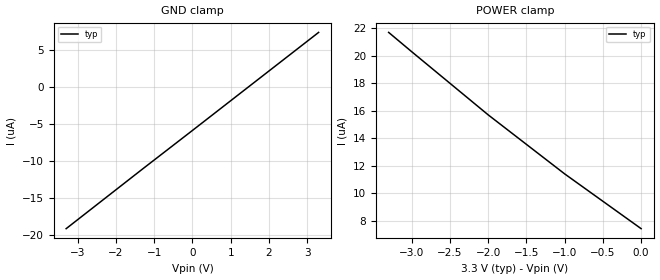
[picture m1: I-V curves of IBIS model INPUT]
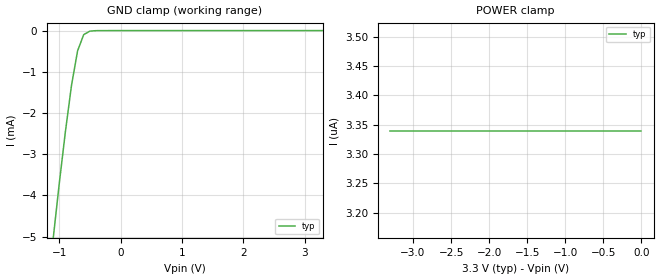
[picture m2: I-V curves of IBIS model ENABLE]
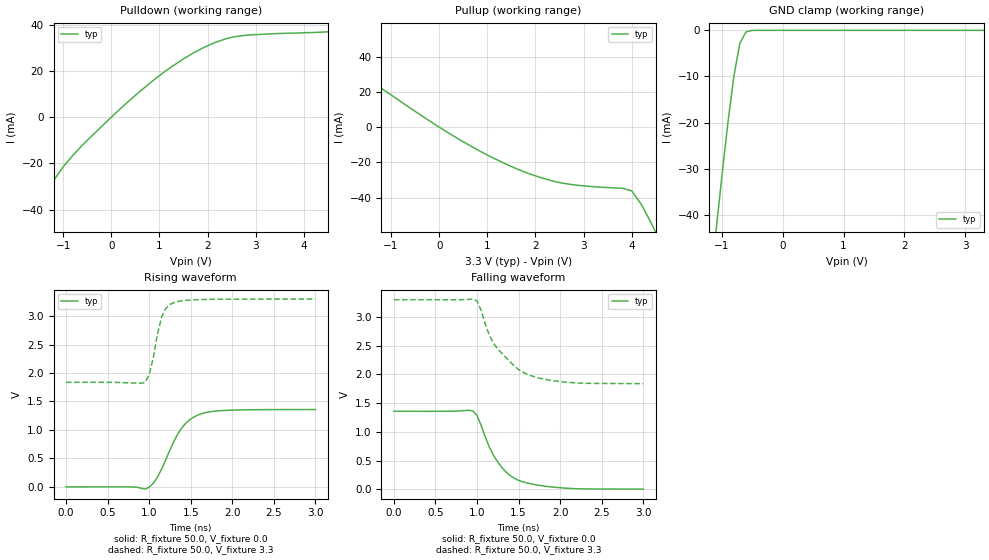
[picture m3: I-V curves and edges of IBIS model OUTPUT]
|   Texas Instruments Incorporated
|   Data Transmissions Products
|   IBIS Model for SN65LVDS352
|   24PW TSSOP Package
[IBIS Ver]   3.2
[Comment char]   |_char
[File name]   lvds352.ibs
[File Rev]   1.0
[Date]   23Aug01
[Source]   File originated at Texas Instruments Incorporated.
   Data Transmission Products Group. All data based on
   Bench Measurements.
[Notes]
[Disclaimer]
(C) Copyright Texas Instruments Incorporated 2001
   All rights reserved
  Texas Instruments Incorporated hereby grants the user of this IBIS
model a non-exclusive, nontransferable license to use this IBIS model
under the following terms.  Before using this IBIS model, the user
should read this license.  If the user does not accept these terms,
the IBIS model should be returned to Texas Instruments within 30 days.
  The user is granted this license only to use the IBIS model and
is not granted rights to sell, load, rent, lease or license the IBIS
model in whole or in part, or in modified form to anyone other than
user.  User may modify the IBIS model to suit its specific applications
but rights to derivative works and such modifications shall belong to
Texas Instruments.
  This IBIS model is provided on an "AS IS" basis and Texas Instruments
makes absolutely no warranty with respect to the information contained
herein.  TEXAS INSTRUMENTS DISCLAIMS AND CUSTOMER WAIVES ALL WARRANTIES,
EXPRESS OR IMPLIED, INCLUDING WARRANTIES OF MERCHANTABILITY OR FITNESS
FOR A PARTICULAR PURPOSE. The entire risk as to quality and performance
is with the Customer. ACCORDINGLY, IN NO EVENT SHALL THE COMPANY BE LIABLE
FOR ANY DAMAGES, WHETHER IN CONTRACT OR TORT,INCLUDING ANY LOST PROFITS
OR OTHER INCIDENTAL, CONSEQUENTIAL, EXEMPLARY, OR PUNITIVE DAMAGES ARISING
OUT OF THE USE OR APPLICATION OF THE IBIS model provided in this package.
Further, Texas Instruments reserves the right to discontinue or make changes
without notice to any product herein to improve reliability, function, or
design. Texas Instruments does not convey any license under patent rights
or any other intellectual property rights, including those of third parties.
Contact Texas Instruments at ATTN:DATA TRANSMISSIONS
[Copyright]   Copyright 2001, Texas Instruments, All Rights Reserved
[Component]   SN65LVDS352PW
[Manufacturer]  Texas Instruments Incorporated
[Package]
|   typ   min   max
R_pkg   0.039   0.030   0.046
L_pkg   2.685nH   2.367nH   3.177nH
C_pkg   0.320pF   0.252pF   0.434pF
[Pin]   signal_name   model_name   R_pin   L_pin   C_pin
1   1A   INPUT   0.037   3.153n   0.434p
2   1B   INPUT   0.034   2.629n   0.341p
3   2A   INPUT   0.032   2.860n   0.347p
4   2B   INPUT   0.042   2.741n   0.290p
5   EN1,2   ENABLE   0.046   2.600n   0.262p
6   VCC   POWER   0.043   2.414n   0.266p
7   GND   GND   0.042   2.367n   0.262p
8   EN3,4   ENABLE   0.044   2.461n   0.252p
9   3A   INPUT   0.042   2.543n   0.274p
10   3B   INPUT   0.030   2.616n   0.332p
11   4A   INPUT   0.037   2.670n   0.346p
12   4B   INPUT   0.039   3.177n   0.433p
13   /FS4   NC
14   4Y   OUTPUT   0.037   2.656n   0.345p
15   DGND2   GND   0.031   2.739n   0.340p
16   VCCD2   POWER   0.042   2.649n   0.282p
17   3Y   OUTPUT   0.046   2.532n   0.257p
18   /FS3   NC
19   /FS2   NC
20   2Y   OUTPUT   0.046   2.532n   0.257p
21   VCCD1   POWER   0.042   2.648n   0.282p
22   DGND1   GND   0.031   2.738n   0.339p
23   1Y   OUTPUT   0.036   2.653n   0.344p
24   /FS1   NC
[Diff_pin]   inv_pin   vdiff   tdelay_typ   tdelay_min   tdelay_max
| The 'xA' pin is Diff_pin and the 'xB' pin is the inv_pin
2   1   50mV   0 0 0   | Vth  +/-50mV
6   7   50mV   0 0 0
10   9   50mV   0 0 0
14   15   50mV   0 0 0
| Models and submodels in the file (3): INPUT (Input), ENABLE (Input), OUTPUT (3-state)
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|   Receiver Input Model
[Model]   INPUT
Model_type   Input
|Signals   1A,1B,2A,2B,3A,3B,4A,4B
Vinh = 2.0
Vinl = 0.8
|   typ   min   max
C_comp   1.0pF   NA   NA
|   typ   min   max
[Temperature Range]   25.0   NA   NA
[Voltage range]   3.3V   3.0V   3.6V
[GND_clamp]
|   Voltage   I(typ)   I(min)   I(max)
-3.3V     -19.2uA    NA         NA
-1.3V     -11.1uA    NA         NA
0V        -5.89uA    NA         NA
1.3V      -651nA     NA         NA
3.3V      7.41uA     NA         NA
[Power_clamp]
| Note that the[POWER_clamp]voltage table is referenced to Vcc
| and is calculated using Vtable=Vcc - Vmeasured.
|   Voltage   I(typ)   I(min)   I(max)
-3.3V     21.7uA     NA         NA
-3V       20.3uA     NA         NA
-2V       15.7uA     NA         NA
-1V       11.4uA     NA         NA
0V        7.41uA     NA         NA
|   Receiver Enable Model
[Model]   ENABLE
Model_type   Input
|Signals   EN1,2 EN3,4
Vinh = 2.0
Vinl = 0.8
|   typ   min   max
C_comp   1.0pF   NA   NA
|   typ   min   max
[Temperature Range]   25.0   NA   NA
[Voltage range]   3.3V   3.0V   3.6V
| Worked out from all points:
|   GND clamp passes 1 mA (typ) near -0.76 V on its own axis
[GND_clamp]
|   Voltage   I(typ)   I(min)   I(max)
-3.3V     -43.1mA    NA         NA
-1.1V     -5.08mA    NA         NA
-1V       -3.73mA    NA         NA
-900mV    -2.47mA    NA         NA
-800mV    -1.34mA    NA         NA
-700mV    -493uA     NA         NA
-600mV    -98.5uA    NA         NA
-500mV    -13.3uA    NA         NA
3.3V      3.34pA     NA         NA
[Power_clamp]
| Note that the[POWER_clamp]voltage table is referenced to Vcc
| and is calculated using Vtable=Vcc - Vmeasured.
|   Voltage   I(typ)   I(min)   I(max)
-3.3V     3.34uA     NA         NA
-2.7V     3.34uA     NA         NA
-2V       3.34uA     NA         NA
-800mV    3.34uA     NA         NA
0V        3.34uA     NA         NA
|   Receiver Output Model
[Model]   OUTPUT
Model_type   3-state
| Signals   1Y,2Y,3Y,4Y
Vmeas = 1.5V   |Reference voltage for timing measurements
Cref = 8pF   |Timing specification test load capacitance value
Vref = 0   |Timing specification test load voltage; GND
| variable   typ   min   max
C_comp   1.0pF   NA   NA
|   typ   min   max
[Temperature Range]   25.0   NA   NA
[Voltage range]   3.3V   3.0V   3.6V
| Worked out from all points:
|   slope of the pulldown table from 0 to 0.495 V, typ, clamps not added: 52.7 ohm
|   slope of the pullup table from 0 to 0.495 V, typ, clamps not added: 60.3 ohm
|   GND clamp passes 1 mA (typ) near -0.63 V on its own axis
|   rising waveform, R_fixture 50.0, V_fixture 0.0: 20-80 % time 287ps typ, NA min, NA max; typ from 0.001 V to 1.36 V
|   falling waveform, R_fixture 50.0, V_fixture 0.0: 20-80 % time 315ps typ, NA min, NA max; typ from 1.36 V to 0.004 V
|   rising waveform, R_fixture 50.0, V_fixture 3.3: 20-80 % time 131ps typ, NA min, NA max; typ from 1.84 V to 3.3 V
|   falling waveform, R_fixture 50.0, V_fixture 3.3: 20-80 % time 389ps typ, NA min, NA max; typ from 3.3 V to 1.84 V
[Pulldown]
|   Voltage   I(typ)   I(min)   I(max)
-3.3V     -150mA     NA         NA
-1.6V     -47.9mA    NA         NA
-1.2V     -27.5mA    NA         NA
-1V       -21.5mA    NA         NA
-600mV    -12.1mA    NA         NA
200mV     3.91mA     NA         NA
900mV     16.4mA     NA         NA
1.5V      25.3mA     NA         NA
2.1V      31.9mA     NA         NA
2.5V      34.6mA     NA         NA
2.9V      35.7mA     NA         NA
6.6V      39.1mA     NA         NA
[Pullup]
|   Voltage   I(typ)   I(min)   I(max)
| Note that the[Pullup]voltage table is referenced to Vcc
| and is calculated using Vtable=Vcc - Vmeasured.
-3.3V     61mA       NA         NA
-3.1V     57.2mA     NA         NA
-3V       55.4mA     NA         NA
100mV     -1.72mA    NA         NA
900mV     -14.4mA    NA         NA
1.6V      -23.5mA    NA         NA
2.5V      -31.4mA    NA         NA
4V        -36.1mA    NA         NA
4.2V      -43.8mA    NA         NA
4.4V      -54.1mA    NA         NA
4.6V      -65.3mA    NA         NA
6.6V      -187mA     NA         NA
| Output in High Impedance (off)
[GND_clamp]
|   Voltage   I(typ)   I(min)   I(max)
-3.3V     -347mA     NA         NA
-1.1V     -44.7mA    NA         NA
-1V       -32.3mA    NA         NA
-900mV    -20.5mA    NA         NA
-800mV    -10.1mA    NA         NA
-700mV    -2.82mA    NA         NA
-600mV    -350uA     NA         NA
-500mV    -29.4uA    NA         NA
-400mV    -1.91uA    NA         NA
3.3V      426pA      NA         NA
[POWER_clamp]
|   Voltage   I(typ)   I(min)   I(max)
| Note that the [POWER_clamp] voltage table is referenced to Vcc
| and is calculated using Vtable = Vcc - Vmeasured.
| Outputs in Tri-state.
-3.3V     0A         NA         NA
0V        0A         NA         NA
[Ramp]
|   typ   min   max
dV/dt_r   0.815V/389ps   NA   NA
dV/dt_f   0.880V/285ps   NA   NA
R_load = 50
[Rising Waveform]
R_fixture = 50.0
V_fixture = 0.0
C_fixture = 0p
L_fixture = 0n
|   V(typ)   V(min)   V(max)
0s        1mV        NA         NA
950ps     -39mV      NA         NA
1ns       -5mV       NA         NA
1.1ns     171mV      NA         NA
1.3ns     807mV      NA         NA
1.4ns     1.051V     NA         NA
1.5ns     1.192V     NA         NA
1.65ns    1.295V     NA         NA
2.05ns    1.351V     NA         NA
3ns       1.359V     NA         NA
[Falling Waveform]
R_fixture = 50.0
V_fixture = 0.0
C_fixture = 0p
L_fixture = 0n
|   V(typ)   V(min)   V(max)
0s        1.359V     NA         NA
950ps     1.365V     NA         NA
1ns       1.285V     NA         NA
1.15ns    728mV      NA         NA
1.25ns    474mV      NA         NA
1.4ns     239mV      NA         NA
1.55ns    132mV      NA         NA
1.8ns     59mV       NA         NA
2.05ns    23mV       NA         NA
3ns       4mV        NA         NA
[Rising Waveform]
R_fixture = 50.0
V_fixture = 3.3
C_fixture = 0p
L_fixture = 0n
|   V(typ)   V(min)   V(max)
0s        1.836V     NA         NA
950ps     1.834V     NA         NA
1ns       1.971V     NA         NA
1.05ns    2.27V      NA         NA
1.1ns     2.682V     NA         NA
1.15ns    2.984V     NA         NA
1.2ns     3.135V     NA         NA
1.3ns     3.238V     NA         NA
1.7ns     3.292V     NA         NA
3ns       3.298V     NA         NA
[Falling Waveform]
R_fixture = 50.0
V_fixture = 3.3
C_fixture = 0p
L_fixture = 0n
|   V(typ)   V(min)   V(max)
0s        3.299V     NA         NA
950ps     3.311V     NA         NA
1ns       3.279V     NA         NA
1.05ns    3.109V     NA         NA
1.15ns    2.674V     NA         NA
1.2ns     2.537V     NA         NA
1.45ns    2.144V     NA         NA
1.65ns    1.977V     NA         NA
2.1ns     1.862V     NA         NA
3ns       1.84V      NA         NA
